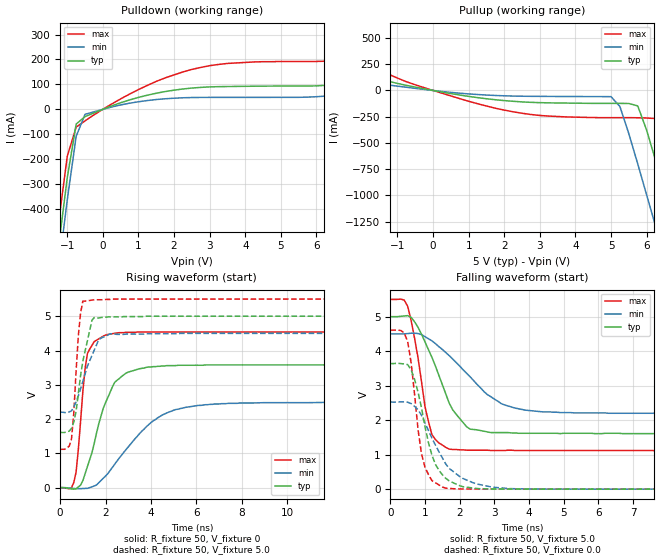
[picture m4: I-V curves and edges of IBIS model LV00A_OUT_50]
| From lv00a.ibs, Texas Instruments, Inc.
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|   Model LV00A_OUT_50
[Model]   LV00A_OUT_50
Model_type  Output
Polarity   Non-Inverting
Vmeas = 2.50v
Cref = 15pf
| variable   typ   min   max
C_comp   4.62pf   3.47pf   5.77pf
[Temperature Range]   25   85   -40
[Voltage Range]   5.0   4.5   5.5
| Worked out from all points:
|   slope of the pulldown table from 0 to 0.75 V, typ, clamps not added: 19.9 ohm
|   slope of the pullup table from 0 to 0.75 V, typ, clamps not added: 17.2 ohm
|   rising waveform, R_fixture 50, V_fixture 0: 20-80 % time 1ns typ, 2.01ns min, 366ps max; typ from 0 V to 3.58 V
|   falling waveform, R_fixture 50, V_fixture 5.0: 20-80 % time 833ps typ, 1.42ns min, 440ps max; typ from 5 V to 1.61 V
|   rising waveform, R_fixture 50, V_fixture 5.0: 20-80 % time 501ps typ, 731ps min, 252ps max; typ from 1.61 V to 5 V
|   falling waveform, R_fixture 50, V_fixture 0.0: 20-80 % time 524ps typ, 868ps min, 330ps max; typ from 3.64 V to 0 V
[Pulldown]
|   Voltage   I(typ)   I(min)   I(max)
-5V       -5.14A     -5.22A     -5.05A
-1.5V     -853mA     -945mA     -756mA
-1.25V    -557mA     -649mA     -461mA
-1V       -274mA     -363mA     -188mA
-750mV    -58.9mA    -108mA     -71.3mA
-500mV    -29.2mA    -20mA      -46.2mA
0V        -3.33nA    -3.4nA     -3.57nA
1.25V     56.7mA     35.2mA     96mA
2.5V      85.3mA     47.3mA     160mA
3.5V      91.4mA     47.8mA     184mA
6.75V     103mA      58.5mA     199mA
10V       179mA      107mA      329mA
[Pullup]
|   Voltage   I(typ)   I(min)   I(max)
-5V       317mA      173mA      595mA
-3.5V     253mA      144mA      466mA
-750mV    48.6mA     30.8mA     83.5mA
1.5V      -78.8mA    -43.5mA    -148mA
5V        -123mA     -58.9mA    -259mA
5.25V     -123mA     -153mA     -259mA
5.75V     -147mA     -699mA     -260mA
6.25V     -664mA     -1.29A     -268mA
6.5V      -960mA     -1.6A      -403mA
6.75V     -1.26A     -1.9A      -685mA
7.25V     -1.87A     -2.51A     -1.28A
10V       -5.25A     -5.89A     -4.66A
[Ramp]
| variable   typ   min   max
dV/dt_r   2.15E+00/9.41E-10   1.50E+00/2.01E-09   2.72E+00/3.55E-10
dV/dt_f   2.05E+00/8.21E-10   1.40E+00/1.40E-09   2.64E+00/4.81E-10
R_load = 50
[Rising Waveform]
R_fixture = 50
V_fixture = 0
|   Time   V(typ)   V(min)   V(max)
0s        0V         0V         0V
500ps     -35.4mV    -18.3mV    393uV
700ps     -30.7mV    -26.9mV    446mV
1ns       206mV      -24.2mV    2.81V
1.2ns     614mV      -18.7mV    3.91V
2.1ns     2.63V      410mV      4.47V
2.9ns     3.34V      1.11V      4.53V
4.1ns     3.53V      1.95V      4.54V
6.1ns     3.57V      2.4V       4.54V
25ns      3.58V      2.49V      4.54V
[Falling Waveform]
R_fixture = 50
V_fixture = 5.0
V_fixture_min = 4.5
V_fixture_max = 5.5
|   Time   V(typ)   V(min)   V(max)
0s        5V         4.5V       5.5V
500ps     5.03V      4.51V      5.3V
800ps     4.69V      4.51V      3.8V
1ns       4.27V      4.42V      2.39V
1.2ns     3.82V      4.3V       1.58V
1.7ns     2.49V      3.87V      1.16V
2.3ns     1.74V      3.26V      1.13V
3.2ns     1.64V      2.48V      1.12V
4.4ns     1.62V      2.24V      1.12V
25ns      1.61V      2.2V       1.12V
[Rising Waveform]
R_fixture = 50
V_fixture = 5.0
V_fixture_min = 4.5
V_fixture_max = 5.5
|   Time   V(typ)   V(min)   V(max)
0s        1.61V      2.2V       1.12V
500ps     1.73V      2.24V      1.42V
600ps     1.91V      2.35V      2.17V
800ps     2.74V      2.68V      4.43V
900ps     3.27V      2.88V      5.1V
1ns       3.69V      3.1V       5.44V
1.4ns     4.88V      3.85V      5.47V
1.7ns     4.95V      4.32V      5.48V
2.2ns     4.98V      4.49V      5.49V
25ns      5V         4.5V       5.5V
[Falling Waveform]
R_fixture = 50
V_fixture = 0.0
|   Time   V(typ)   V(min)   V(max)
0s        3.64V      2.53V      4.61V
500ps     3.61V      2.52V      4.28V
600ps     3.46V      2.48V      3.66V
800ps     2.81V      2.3V       1.72V
1ns       1.81V      1.92V      631mV
1.3ns     719mV      1.28V      186mV
1.6ns     314mV      729mV      29.5mV
2.4ns     31.7mV     181mV      3.57mV
3.5ns     2.96mV     14.9mV     1.27mV
25ns      8.53uV     1.52uV     9.61uV
